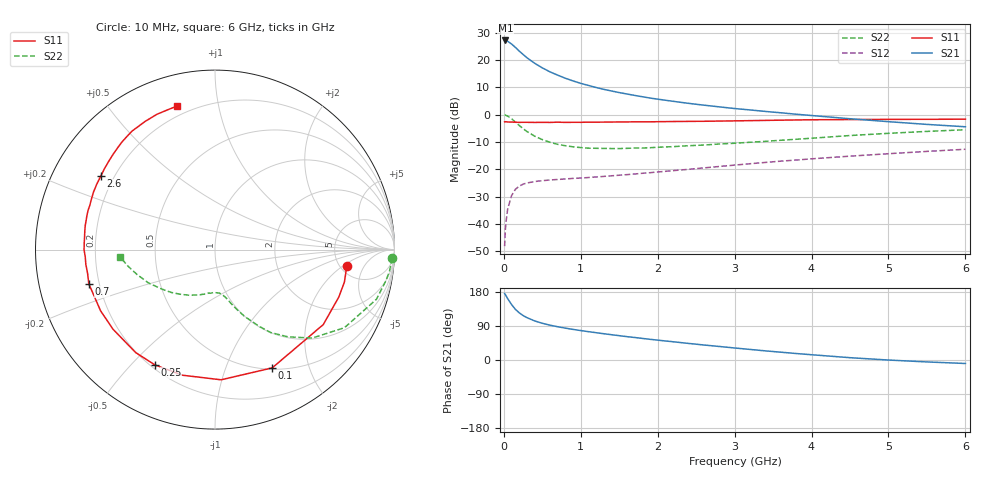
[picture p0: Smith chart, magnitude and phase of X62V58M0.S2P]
! SIEMENS Small Signal Semiconductors
! BFP193W
! Si NPN RF Bipolar Junction Transistor in SOT343
! VCE = 2.5 V  IC = 8 mA
! Common Emitter S-Parameters:  April 1994
# GHz  S  MA  R  50
!  f  S11  S21  S12  S22
! GHz  MAG  ANG  MAG  ANG  MAG  ANG  MAG  ANG
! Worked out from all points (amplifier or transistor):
!   40 points, 10 MHz to 6 GHz, reference 50 ohm
!   highest |S21| = 27.2 dB at 20 MHz (marker M1)
!   |S21| within 3 dB of that: start of sweep to 167.1 MHz
!   unconditionally stable (mu >= 1): 1.412 GHz to 4.208 GHz
!   at 200 MHz: K = 0.19, MSG = 24.7 dB, |S12| = -26.2 dB
!   at 1.5 GHz: K = 1.03, MAG = 14.0 dB, |S12| = -22.2 dB
!   at 6 GHz: K = 0.93, MSG = 4.1 dB, |S12| = -12.7 dB
!   lowest NFmin = 1.25 dB at 450 MHz
!   S11 on the Smith chart (normalised r, x): 10 MHz: 5.78, -2.27; 100 MHz: 0.52, -1.47; 250 MHz: 0.22, -0.58; 700 MHz: 0.16, -0.13; 2.6 GHz: 0.15, +0.29; 6 GHz: 0.15, +0.76
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0.01  0.7402 -6.9  22.81 175.5  0.0039 86.6  0.9872 -2.7
0.02  0.7434 -14.1  22.87 172.6  0.0079 82.9  0.9797 -7.1
0.03  0.7386 -21.0  22.64 169.0  0.0113 81.1  0.9676 -10.4
0.05  0.7338 -34.7  22.06 161.8  0.0187 74.6  0.9411 -17.1
0.1  0.732 -64.2  19.7 146.4  0.0328 60.6  0.8424 -31.1
0.15  0.7262 -87.3  17.07 133.8  0.0429 50.7  0.7324 -42.3
0.2  0.7232 -104.7  14.62 124.5  0.049 43.7  0.6335 -50.1
0.25  0.7244 -117.6  12.68 117.4  0.0533 38.6  0.5568 -56.1
0.3  0.7242 -127.6  11.03 111.8  0.056 35.2  0.4914 -60.2
0.4  0.7209 -142.0  8.748 103.2  0.0595 30.8  0.4043 -66.3
0.5  0.723 -151.9  7.197 96.9  0.0618 29.1  0.3492 -70.4
0.6  0.7212 -158.8  6.076 91.9  0.0636 28.1  0.3121 -73.5
0.7  0.7286 -164.8  5.294 87.8  0.065 28.3  0.2861 -75.8
0.9  0.7244 -173.5  4.152 80.7  0.068 29.0  0.2574 -80.2
1.1  0.7295 -179.9  3.429 74.8  0.0706 30.8  0.2436 -84.1
1.6  0.7364 166.9  2.39 61.6  0.0797 35.9  0.2415 -93.7
2.2  0.749 154.7  1.757 48.1  0.0943 40.8  0.2595 -106.0
2.6  0.7565 147.3  1.493 39.6  0.1059 43.0  0.2776 -114.5
3.2  0.7768 137.1  1.221 27.9  0.1262 44.0  0.3122 -126.9
4.5  0.8132 118.7  0.842 6.1  0.1737 41.0  0.4147 -153.4
5.5  0.8219 109.3  0.663 -5.1  0.2123 36.4  0.4934 -169.2
6  0.827 104.9  0.6 -9.2  0.2325 33.9  0.5295 -175.5
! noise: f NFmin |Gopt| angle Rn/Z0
0.45  1.25  0.23  133  0.12
0.9  1.3  0.35  156  0.11
1.8  2  0.55  -155  0.13
